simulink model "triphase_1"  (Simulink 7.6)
settings: Solver=ode15s  StartTime=0.0  StopTime=5/60  RelTol=1e-3
InitFcn:
  | clc
undefined symbols (not defined in the file or in its folder): Angle, Magnitude
libraries: powerlib x9, powerlib_extras x2

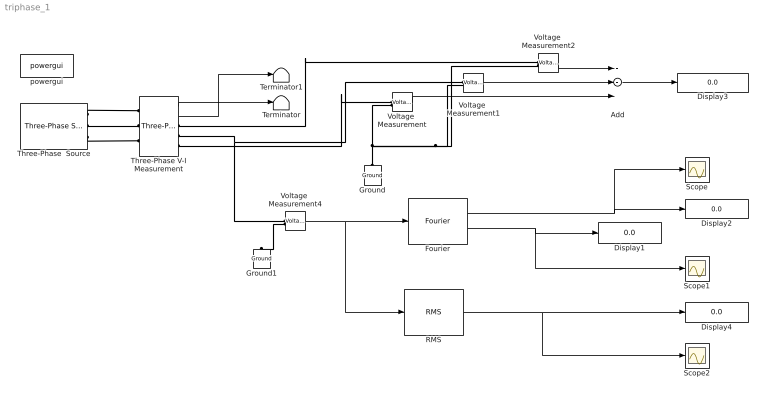
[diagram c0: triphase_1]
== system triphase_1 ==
  Add : Sum  Inputs=+++
  Display{1..4} (4 alike) : Display
  Fourier : powerlib_extras/Measurements/Fourier  DialogController=POWERSYS.PowerSysDialog  SystemSampleTime=-1  f1=60  n=1
  Ground : powerlib/Elements/Ground  DialogController=POWERSYS.PowerSysDialog  PhysicalDomain=powersysdomain  SubClassName=unknown  LeftPortType=p1  RightPortType=p1  LConnTagsString=a
  Ground1 : powerlib/Elements/Ground  DialogController=POWERSYS.PowerSysDialog  PhysicalDomain=powersysdomain  SubClassName=unknown  LeftPortType=p1  RightPortType=p1  LConnTagsString=a
  RMS : powerlib_extras/Measurements/RMS  DialogController=POWERSYS.PowerSysDialog  SystemSampleTime=-1  f1=60
  Scope : Scope
  Scope1 : Scope
  Scope2 : Scope
  Terminator : Terminator
  Terminator1 : Terminator
  Three-Phase V-I Measurement : powerlib/Measurements/Three-Phase V-I Measurement  DialogController=POWERSYS.PowerSysDialog  SystemSampleTime=-1  VoltageMeasurement=phase-to-ground  SetLabelV=off  LabelV=Vabc  Vpu=off  VpuLL=off  CurrentMeasurement=yes  SetLabelI=off  LabelI=Iabc  Ipu=off  Pbase=100e6  Vbase=500e3  OutputType=Magnitude-Angle  PhasorSimulation=off  PSBequivalent=0
  Three-Phase  Source : powerlib/Electrical Sources/Three-Phase Source  DialogController=POWERSYS.PowerSysDialog  SystemSampleTime=-1  Voltage=25e3  PhaseAngle=0  Frequency=60  InternalConnection=Yg  SpecifyImpedance=off  Resistance=0.8929  Inductance=1e-6  ShortCircuitLevel=100e6  BaseVoltage=25e3  XRratio=1e-12
  Voltage  Measurement : powerlib/Measurements/Voltage Measurement  DialogController=POWERSYS.PowerSysDialog  SystemSampleTime=-1  PhasorSimulation=off  OutputType=Complex  PSBequivalent=0
  Voltage  Measurement1 : powerlib/Measurements/Voltage Measurement  DialogController=POWERSYS.PowerSysDialog  SystemSampleTime=-1  PhasorSimulation=off  OutputType=Complex  PSBequivalent=0
  Voltage  Measurement2 : powerlib/Measurements/Voltage Measurement  DialogController=POWERSYS.PowerSysDialog  SystemSampleTime=-1  PhasorSimulation=off  OutputType=Complex  PSBequivalent=0
  Voltage  Measurement4 : powerlib/Measurements/Voltage Measurement  DialogController=POWERSYS.PowerSysDialog  SystemSampleTime=-1  PhasorSimulation=off  OutputType=Magnitude-Angle  PSBequivalent=0
  powergui : powerlib/powergui  Priority=1  SystemSampleTime=-1  SimulationMode=Continuous  SampleTime=50e-6  frequency=60  SPID=off  DisableSnubberDevices=off  DisableRonSwitches=off  DisableVfSwitches=off  SwTol=0  Interpol=off  frequencyindice=60  echomessages=off  HookPort=off  DisplayEquations=off  FunctionMessages=off  EnableUseOfTLC=off  x0status=blocks  RestoreLinks=warning  ResistiveCurrentMeasurement=off  Ylog=off  Xlog=on  ShowGrid=off  save=off  variable=ZData  ZoomFFT=off  StartTime=0.0  cycles=1  DisplayStyle=1  FreqAxis=off  MaxFrequency=1000  frequencyindicesteady=1  display=off  methode=off
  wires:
  Voltage  Measurement2/1 -> Add/1
  Voltage  Measurement1/1 -> Add/2
  Voltage  Measurement/1 -> Add/3
  Add/1 -> Display3/1
  Three-Phase V-I Measurement/1 -> Terminator/1
  Three-Phase V-I Measurement/2 -> Terminator1/1
  Fourier/2 -> Display1/1, Scope1/1
  Fourier/1 -> Display2/1, Scope/1
  Voltage  Measurement4/1 -> Fourier/1, RMS/1
  RMS/1 -> Display4/1, Scope2/1
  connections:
  Voltage  Measurement4/LConn1 -- Three-Phase V-I Measurement/RConn2 -- Voltage  Measurement1/LConn1
  Voltage  Measurement1/LConn2 -- Voltage  Measurement2/LConn2 -- Ground/LConn1 -- Voltage  Measurement/LConn2
  Three-Phase  Source/RConn1 -- Three-Phase V-I Measurement/LConn1
  Three-Phase  Source/RConn2 -- Three-Phase V-I Measurement/LConn2
  Three-Phase  Source/RConn3 -- Three-Phase V-I Measurement/LConn3
  Voltage  Measurement4/LConn2 -- Ground1/LConn1
  Three-Phase V-I Measurement/RConn1 -- Voltage  Measurement2/LConn1
  Three-Phase V-I Measurement/RConn3 -- Voltage  Measurement/LConn1
